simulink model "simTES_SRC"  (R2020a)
settings: Solver=ode15s  StartTime=0.0  StopTime=tsim  MaxStep=1/3600  RelTol=1e-3
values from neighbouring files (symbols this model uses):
  dq = 500    [runTES.m]
  dqS = 500    [runTES.m]
  KcSRC = 1/alpha(1)*1/kp*1/(tauCSRC+thetaSRC)    [runTES.m]
  nd = 1    [runTES.m]    (also in Main.m = size(d0,2); Main_OL.m = size(d0,2); runTestCalcBlk.m = size(d0,2); runTransf.m = size(d0,2))
  np = length(param)    [runTES.m]    (also in runH2Psim.m; Main.m = size(p,2); Main_OL.m = size(p,2); runTestCalcBlk.m = size(p,2))
  nu = 4    [runTES.m]    (also in runH2Psim.m = length(u0); Main.m = 1; Main_OL.m = 1; runTestCalcBlk.m = 1)
  nx = 2    [runTES.m]    (also in H2P_Turbine_driven.m = param(end); runTD.m = length(x0); H2P_Boiler_driven.m = param(end); runBD.m = length(x0))
  param = [V;rho;p0;m0;eps]    [runTES.m]    (also in runTD.m = [Tref;TrefB;dHvap;cpg;cpW;cpSt;R;Mwt;     T0;TG0;ME;pC;     ; runBD.m = [Tref;TrefB;dHvap;cpg;cpW;cpSt;R;Mwt;          T0;TG0;ME;pC;; runFP.m = [Tref;TrefB;dHvap;cpg;cpW;cpSt;R;Mwt;          T0;TG0;ME;pC;; runFPV2.m = [Tref;TrefB;dHvap;cpg;cpW;cpSt;R;Mwt;          T0;TG0;ME;pC;)
  ps = p0    (= 5)    [runTES.m]
  pSR = [u0;alpha;umax;N]    [runTES.m]
  qS0 = qnom    (= 500)    [runTES.m]
  qsp = qnom    (= 500)    [runTES.m]
  tauISRC = 4*(tauCSRC+thetaSRC)    (= 0.0111111111111)    [runTES.m]
  td1 = 1    [runTES.m]
  td2 = 15    [runTES.m]
  tq1 = 12    [runTES.m]
  tq2 = 40    [runTES.m]
  Vmax = V    (= 5000)    [runTES.m]
  x0 = [Vh0;p0]    [runTES.m]    (also in runTD.m = [TE0;TD0;TSh0;MD0; MSh0;w0;TA0;0;0;0;0;0;0;0;0;0]; runBD.m = [TE0;TD0;TSh0;MD0; MSh0;w0;TA0;0;0;0;0;0;0;0;0;0]; runFP.m = [TE0;TD0;TSh0;MD0; MSh0;w0;TA0;0;0;0;0;0;0;0]; runFPV2.m = [TE0;TD0;TSh0;MD0; MSh0;w0;TA0;0;0;0;0;0;0;0])
undefined symbols (not defined in the file or in its folder): ChargingPolicy, TESmodel

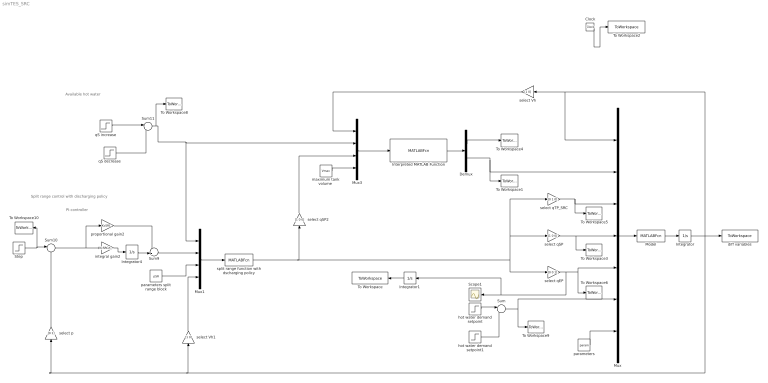
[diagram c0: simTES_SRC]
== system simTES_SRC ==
  note: Available hot water
  note: Split range control with discharging policy
  note: PI-controller
  Clock : Clock
  Demux : Demux  Outputs=2
  Integrator : Integrator  InitialCondition=x0
  Integrator1 : Integrator
  Integrator4 : Integrator
  Interpreted MATLAB Function : MATLABFcn  MATLABFcn=ChargingPolicy(u(1),u(2),u(3),u(4))  OutputDimensions=2
  Model : MATLABFcn  MATLABFcn=TESmodel(u(1:nx),u(nx+1:nx+nu),u(nx+nu+1:nx+nu+nd),u(nx+nu+nd+1:nx+nu+nd+np))  OutputDimensions=nx
  Mux : Mux  Inputs=7
  Mux1 : Mux
  Mux3 : Mux
  Scope1 : Scope
  Step : Step  Before=ps  After=ps  SampleTime=0
  Sum : Sum  Inputs=|+-
  Sum10 : Sum  Inputs=|+-
  Sum11 : Sum  Inputs=|++
  Sum9 : Sum  Inputs=++|
  To Workspace : ToWorkspace  VariableName=JSRC  SampleTime=-1
  To Workspace1 : ToWorkspace  VariableName=qSTSRC  SampleTime=-1
  To Workspace10 : ToWorkspace  VariableName=pref  SampleTime=-1
  To Workspace2 : ToWorkspace  VariableName=tSRC  SampleTime=-1
  To Workspace3 : ToWorkspace  VariableName=qSPSRC  SampleTime=-1
  To Workspace4 : ToWorkspace  VariableName=qDSRC  SampleTime=-1
  To Workspace5 : ToWorkspace  VariableName=qTPSRC  SampleTime=-1
  To Workspace6 : ToWorkspace  VariableName=qEPSRC  SampleTime=-1
  To Workspace8 : ToWorkspace  VariableName=qS  SampleTime=-1
  To Workspace9 : ToWorkspace  VariableName=qref  SampleTime=-1
  diff variables : ToWorkspace  VariableName=ySRC  SampleTime=-1
  hot water demand setpoint : Step  Time=tq1  Before=qsp  After=qsp+dq  SampleTime=0
  hot water demand setpoint1 : Step  Time=tq2  After=dq*1.5  SampleTime=0
  integral gain2 : Gain  Gain=KcSRC/tauISRC  Multiplication=Matrix(K*u)
  "maximum tank volume " : Constant  Value=Vmax
  parameters : Constant  Value=param
  parameters split range block : Constant  Value=pSR
  proportional gain2 : Gain  Gain=KcSRC  Multiplication=Matrix(K*u)
  qS decrease : Step  Time=td2  After=-dqS  SampleTime=0
  qS increase : Step  Time=td1  Before=qS0  After=qS0+dqS  SampleTime=0
  select Vh : Gain  Gain=[1 0]  Multiplication=Matrix(K*u)
  select Vh1 : Gain  Gain=[1 0]  Multiplication=Matrix(K*u)
  select p : Gain  Gain=[0 1]  Multiplication=Matrix(K*u)
  select qEP : Gain  Gain=[0 0 1]  Multiplication=Matrix(K*u)
  select qSP : Gain  Gain=[1 0 0]  Multiplication=Matrix(K*u)
  select qSP2 : Gain  Gain=[1 0 0]  Multiplication=Matrix(K*u)
  select qTP_SRC : Gain  Gain=[0 1 0]  Multiplication=Matrix(K*u)
  split range function with dscharging policy : MATLABFcn  MATLABFcn=SRblock(u(1),u(2),u(3:end-1),u(end))  OutputDimensions=3
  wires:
  Model/1 -> Integrator/1
  Integrator/1 -> Mux/1, select Vh/1, diff variables/1, select p/1, select Vh1/1
  Mux/1 -> Model/1
  Mux1/1 -> split range function with dscharging policy/1
  parameters split range block/1 -> Mux1/3
  integral gain2/1 -> Integrator4/1
  Integrator4/1 -> Sum9/2
  Sum10/1 -> proportional gain2/1, integral gain2/1
  proportional gain2/1 -> Sum9/1
  Sum9/1 -> Mux1/2
  Step/1 -> To Workspace10/1, Sum10/1
  select p/1 -> Sum10/2
  qS increase/1 -> Sum11/1
  Clock/1 -> To Workspace2/1
  qS decrease/1 -> Sum11/2
  Sum/1 -> To Workspace9/1, Mux/6
  Mux3/1 -> Interpreted MATLAB Function/1
  "maximum tank volume "/1 -> Mux3/4
  select qEP/1 -> Integrator1/1, Scope1/1, Mux/5, To Workspace6/1
  Interpreted MATLAB Function/1 -> Demux/1
  Demux/1 -> To Workspace4/1
  Demux/2 -> To Workspace1/1, Mux/2
  select qSP/1 -> Mux/4, To Workspace3/1
  split range function with dscharging policy/1 -> select qSP2/1, select qSP/1, select qTP_SRC/1, select qEP/1
  select qSP2/1 -> Mux3/3
  parameters/1 -> Mux/7
  select qTP_SRC/1 -> To Workspace5/1, Mux/3
  select Vh/1 -> Mux3/1
  Sum11/1 -> To Workspace8/1, Mux3/2, Mux1/1
  select Vh1/1 -> Mux1/4
  hot water demand setpoint/1 -> Sum/1
  hot water demand setpoint1/1 -> Sum/2
  Integrator1/1 -> To Workspace/1
